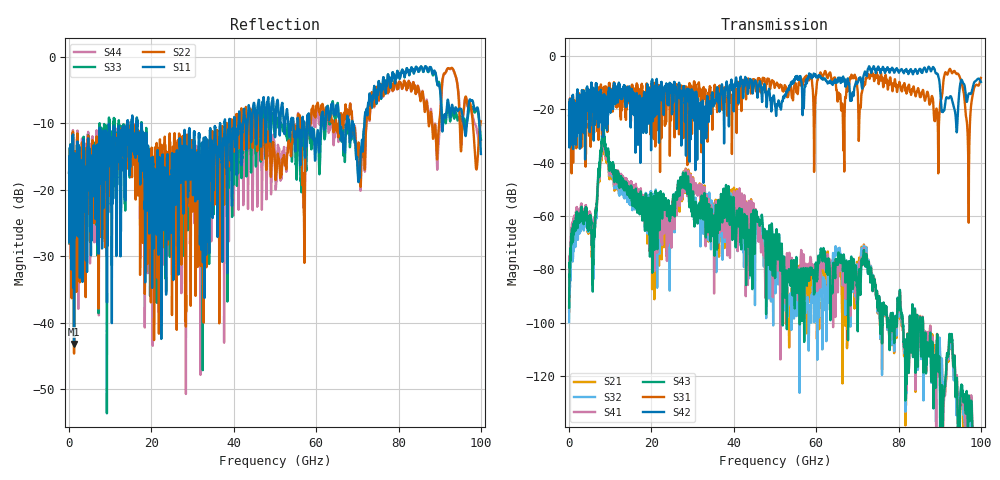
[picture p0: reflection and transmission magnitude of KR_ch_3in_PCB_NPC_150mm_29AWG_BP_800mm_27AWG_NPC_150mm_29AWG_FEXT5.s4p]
# GHz S RI R 45
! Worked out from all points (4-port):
!   4000 points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, 25 MHz to 100 GHz, reference 45 ohm
!   strongest paths, dB at 25 MHz, 25.02 GHz, 50.02 GHz, 75.03 GHz, 100 GHz:
!     S42: -22.2, -20.8, -18.7, -4.1, -9.8
!     S31: -22.2, -12.0, -11.6, -7.8, -8.3
!     S43: -94.3, -58.4, -83.2, -93.3, -154.9
!     S41: -91.8, -60.0, -76.0, -93.5, -147.1
!     S32: -99.7, -63.0, -80.2, -94.2, -161.0
!     S21: -95.8, -56.9, -77.9, -94.4, -158.8
!   lowest |S11| = -43.2 dB at 1.225 GHz (marker M1), VSWR 1.01, Z = 44.9 - j0.619 ohm
!   |S11| at or under -10 dB: start of sweep to 14.14 GHz; 16.58 GHz to 36.66 GHz (20.08 GHz wide, 75.4 % of centre); 68.85 GHz to 71.74 GHz (2.898 GHz wide, 4.12 % of centre)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
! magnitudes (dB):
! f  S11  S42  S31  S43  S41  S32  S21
! 25 MHz  -17.4  -22.2  -22.2  -94.3  -91.8  -99.7  -95.8
! 1.225 GHz  -43.2  -25.9  -25.3  -63.2  -61.0  -68.1  -64.8
! 5.95 GHz  -16.4  -13.6  -14.2  -71.6  -62.4  -73.0  -72.6
! 8.375 GHz  -22.7  -21.4  -18.3  -26.4  -28.0  -27.8  -29.6
! 24.07 GHz  -23.4  -16.0  -15.1  -54.3  -61.5  -58.4  -60.3
! 96.92 GHz  -7.8  -14.7  -37.7  -136.3  -133.8  -142.8  -138.8
! 100 GHz  -14.6  -9.8  -8.3  -154.9  -147.1  -161.0  -158.8
